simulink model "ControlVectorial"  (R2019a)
settings: Solver=VariableStepAuto  StartTime=0.0  StopTime=0.04  RelTol=1e-3
libraries: powerlib x14, eeTransforms x1, powerlib_meascontrol x1, simulink x1

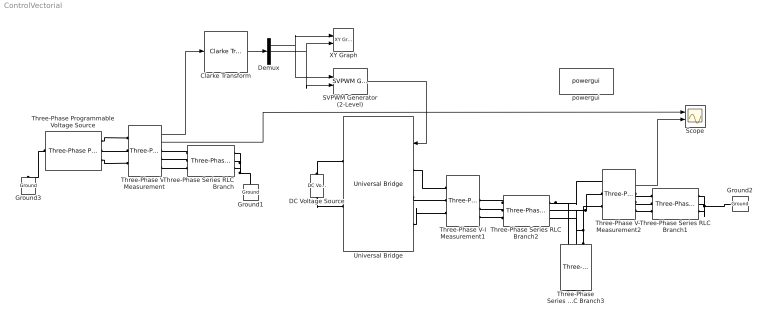
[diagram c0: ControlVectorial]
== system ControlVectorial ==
  Clarke Transform : eeTransforms/Clarke Transform  PowerInvariant=off
  DC Voltage Source : powerlib/Electrical Sources/DC Voltage Source  Amplitude=220*sqrt(2)  Measurements=None
  Demux : Demux  Outputs=3
  Ground1 : powerlib/Elements/Ground  LConnTagsString=a
  Ground2 : powerlib/Elements/Ground  LConnTagsString=a
  Ground3 : powerlib/Elements/Ground  LConnTagsString=a
  SVPWM Generator (2-Level) : powerlib_meascontrol/Pulse & Signal Generators/SVPWM Generator (2-Level)  InputType=alpha-beta components  SwitchingPattern=Pattern #1  Fc=2000  ParUref=[0.8 -30 50]  Ts=0
  Scope : Scope  NumInputPorts=2
  Three-Phase Programmable Voltage Source : powerlib/Electrical Sources/Three-Phase Programmable Voltage Source  PositiveSequence="[220  0 50]"  VariationEntity=None  VariationType=Table of time-amplitude pairs  VariationTypeAlt=Step  VariationStep=0.5  VariationRate=10  VariationMagnitude=0.3  VariationFrequency=2  VariationTiming=[1 2]  VariationPhaseA=off  Amplitudes=[1 0.8 1.2 1.0]  TimeValues=[0 0.1 0.15 0.2]  HarmonicGeneration=off  HarmonicA=[3 0.2 -25 0]  HarmonicB=[2 0.15 35 2]  Timing="[0.05  3]"  BusType=swing  Pref=0  Qref=0  Qmin=-inf  Qmax=inf
  Three-Phase Series RLC Branch : powerlib/Elements/Three-Phase Series RLC Branch  LConnTagsString=A|B|C  RConnTagsString=A|B|C  BranchType=R  Resistance=1  Inductance=1e-3  Capacitance=1e-6  Measurements=None
  Three-Phase Series RLC Branch1 : powerlib/Elements/Three-Phase Series RLC Branch  LConnTagsString=A|B|C  RConnTagsString=A|B|C  BranchType=R  Resistance=1  Inductance=1e-3  Capacitance=1e-6  Measurements=None
  Three-Phase Series RLC Branch2 : powerlib/Elements/Three-Phase Series RLC Branch  LConnTagsString=A|B|C  RConnTagsString=A|B|C  BranchType=L  Resistance=1  Inductance=300e-6*1  Capacitance=1e-6  Measurements=None
  Three-Phase Series RLC Branch3 : powerlib/Elements/Three-Phase Series RLC Branch  LConnTagsString=A|B|C  RConnTagsString=A|B|C  BranchType=C  Resistance=1  Inductance=1e-3  Capacitance=100e-6  Measurements=None
  Three-Phase V-I Measurement : powerlib/Measurements/Three-Phase V-I Measurement  VoltageMeasurement=phase-to-ground  SetLabelV=off  LabelV=Vabc  Vpu=off  VpuLL=off  CurrentMeasurement=yes  SetLabelI=off  LabelI=Iabc  Ipu=off  Pbase=100e6  Vbase=500e3  OutputType=Complex  PhasorSimulation=off  PSBequivalent=0
  Three-Phase V-I Measurement1 : powerlib/Measurements/Three-Phase V-I Measurement  VoltageMeasurement=phase-to-ground  SetLabelV=off  LabelV=Vabc  Vpu=off  VpuLL=off  CurrentMeasurement=yes  SetLabelI=off  LabelI=Iabc  Ipu=off  Pbase=100e6  Vbase=500e3  OutputType=Complex  PhasorSimulation=off  PSBequivalent=0
  Three-Phase V-I Measurement2 : powerlib/Measurements/Three-Phase V-I Measurement  VoltageMeasurement=phase-to-ground  SetLabelV=off  LabelV=Vabc  Vpu=off  VpuLL=off  CurrentMeasurement=yes  SetLabelI=off  LabelI=Iabc  Ipu=off  Pbase=100e6  Vbase=500e3  OutputType=Complex  PhasorSimulation=off  PSBequivalent=0
  Universal Bridge : powerlib/Power Electronics/Universal Bridge  Arms=3  SnubberResistance=1e5  SnubberCapacitance=inf  Device=IGBT / Diodes  Ron=1e-3  Lon=0  ForwardVoltages="[  0  0  ]"  ForwardVoltage=0  GTOparameters=[ 10e-6 , 20e-6 ]  IGBTparameters=[ 1e-6 , 2e-6 ]  Measurements=None  Measurements_2=None  converterType=Rectifier
  XY Graph : simulink/Sinks/XY Graph  xmin=-220  xmax=220  ymin=-220  ymax=220  st=-1
  powergui : powerlib/powergui  Priority=1  SimulationMode=Discrete  SampleTime=50e-7  frequency=50  Iterations=50  frequencyindice=0  Pbase=100e6  ErrMax=1e-4  UnitsV=kV  UnitsW=MW  buscounter=0  FunctionMessages=off  echomessages=off  EnableUseOfTLC=off  CurrentSourceSwitches=off  DisableSnubberDevices=off  DisableRonSwitches=off  DisableVfSwitches=off  DisplayEquations=off  AutomaticDiscreteSolvers=off  SolverType=Tustin/Backward Euler (TBE)  Interpol=off  ExternalGateDelay=off  methode=off  Ts=100  x0status=blocks  SPID=on  SwTol=0  HookPort=off  NonlinearTolerance=0  nMaxIteration=15  ContinueOnMaxIteration=off  RestoreLinks=warning  ResistiveCurrentMeasurement=off  Frange=[0:2:500]  Ylog=off  Xlog=on  ShowGrid=off  save=off  variable=ZData  structure=0  ZoomFFT=off  StartTime=0.0  cycles=1  DisplayStyle=1  fundamental=60  FreqAxis=off  MaxFrequency=1000  frequencyindicesteady=1  RmsSteady=1  display=off
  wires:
  Three-Phase V-I Measurement/1 -> Clarke Transform/1
  Clarke Transform/1 -> Demux/1
  Demux/1 -> XY Graph/1, SVPWM Generator (2-Level)/1
  Demux/2 -> SVPWM Generator (2-Level)/2, XY Graph/2
  SVPWM Generator (2-Level)/1 -> Universal Bridge/1
  Three-Phase V-I Measurement2/2 -> Scope/2
  Three-Phase V-I Measurement/2 -> Scope/1
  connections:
  Three-Phase Series RLC Branch/LConn1 -- Three-Phase V-I Measurement/RConn1
  Three-Phase Series RLC Branch/LConn2 -- Three-Phase V-I Measurement/RConn2
  Three-Phase V-I Measurement/RConn3 -- Three-Phase Series RLC Branch/LConn3
  Three-Phase Programmable Voltage Source/RConn1 -- Three-Phase V-I Measurement/LConn1
  Three-Phase Programmable Voltage Source/RConn2 -- Three-Phase V-I Measurement/LConn2
  Three-Phase Programmable Voltage Source/RConn3 -- Three-Phase V-I Measurement/LConn3
  Three-Phase Series RLC Branch/RConn1 -- Three-Phase Series RLC Branch/RConn2 -- Ground1/LConn1 -- Three-Phase Series RLC Branch/RConn3
  Three-Phase Series RLC Branch1/RConn1 -- Ground2/LConn1 -- Three-Phase Series RLC Branch1/RConn3 -- Three-Phase Series RLC Branch1/RConn2
  Three-Phase Series RLC Branch2/LConn1 -- Three-Phase V-I Measurement1/RConn1
  Three-Phase Series RLC Branch2/LConn2 -- Three-Phase V-I Measurement1/RConn2
  Three-Phase Series RLC Branch2/LConn3 -- Three-Phase V-I Measurement1/RConn3
  Three-Phase Series RLC Branch2/RConn1 -- Three-Phase V-I Measurement2/LConn1 -- Three-Phase Series RLC Branch3/LConn1
  Three-Phase V-I Measurement2/RConn3 -- Three-Phase Series RLC Branch1/LConn3
  Three-Phase Series RLC Branch3/RConn1 -- Three-Phase Series RLC Branch3/RConn2 -- Three-Phase Series RLC Branch3/RConn3
  Three-Phase V-I Measurement2/RConn1 -- Three-Phase Series RLC Branch1/LConn1
  Three-Phase V-I Measurement2/LConn2 -- Three-Phase Series RLC Branch3/LConn2 -- Three-Phase Series RLC Branch2/RConn2
  Three-Phase V-I Measurement2/RConn2 -- Three-Phase Series RLC Branch1/LConn2
  Three-Phase Series RLC Branch3/LConn3 -- Three-Phase V-I Measurement2/LConn3 -- Three-Phase Series RLC Branch2/RConn3
  DC Voltage Source/RConn1 -- Universal Bridge/RConn1
  DC Voltage Source/LConn1 -- Universal Bridge/RConn2
  Universal Bridge/LConn1 -- Three-Phase V-I Measurement1/LConn1
  Universal Bridge/LConn2 -- Three-Phase V-I Measurement1/LConn2
  Universal Bridge/LConn3 -- Three-Phase V-I Measurement1/LConn3
  Three-Phase Programmable Voltage Source/LConn1 -- Ground3/LConn1
